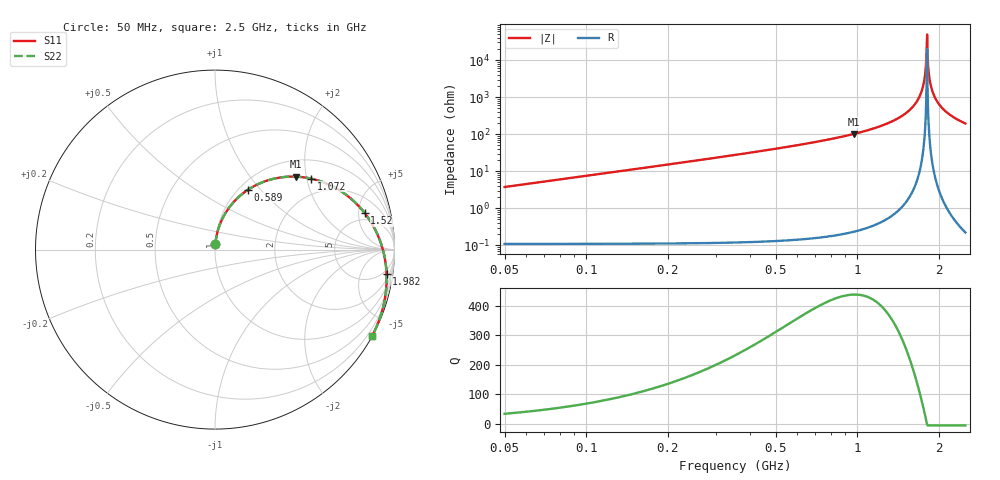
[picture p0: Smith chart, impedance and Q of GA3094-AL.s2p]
! Coilcraft GA3094-AL Air Core Inductor
! 01 July 2008
# MHZ S MA R 50
!Freq  MagS11  AngS11  MagS21  AngS21  MagS12  AngS12  MagS22  AngS22
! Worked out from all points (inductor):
!   351 points, 50 MHz to 2.5 GHz, reference 50 ohm
!   read as 1/Y11, port 2 shorted: L = 12 nH near 57 MHz
!   highest Q = 437 at 967 MHz (marker M1), where L = 16.7 nH
!   self-resonance near 1.8 GHz
!   S11 on the Smith chart (normalised r, x): 50 MHz: 1.00, +0.07; 589 MHz: 1.10, +0.86; 1.072 GHz: 1.50, +2.12; 1.52 GHz: 3.82, +5.92; 1.982 GHz: 3, -13; 2.5 GHz: 0.01, -3.91
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50  0.03286 85.7  0.9984 -2.4  0.9984 -2.4  0.03288 85.7
78  0.05124 85.0  0.9976 -3.8  0.9976 -3.8  0.05127 85.0
106  0.06962 84.0  0.9965 -5.1  0.9965 -5.1  0.06966 84.0
141  0.09258 82.5  0.9946 -6.8  0.9946 -6.8  0.09264 82.5
183  0.1201 80.6  0.9917 -8.9  0.9917 -8.9  0.1202 80.6
239  0.1568 78.0  0.9865 -11.6  0.9865 -11.6  0.1569 78.0
302  0.1979 75.0  0.9791 -14.6  0.9791 -14.6  0.198 75.0
463  0.3021 67.2  0.9521 -22.6  0.9521 -22.6  0.3023 67.2
589  0.3824 61.0  0.9228 -28.8  0.9228 -28.8  0.3826 61.0
869  0.5529 46.9  0.832 -43.0  0.832 -43.0  0.5532 46.9
967  0.6087 41.9  0.7921 -48.0  0.7921 -48.0  0.609 41.9
1072  0.6653 36.5  0.7452 -53.4  0.7452 -53.4  0.6657 36.5
1275  0.7636 26.0  0.6442 -63.9  0.6442 -63.9  0.764 26.0
1520  0.8589 13.7  0.5105 -76.2  0.5105 -76.2  0.8594 13.7
1688  0.9082 5.5  0.4165 -84.4  0.4165 -84.4  0.9087 5.5
1982  0.9652 -8.0  0.2589 -97.9  0.2589 -97.9  0.9657 -8.0
2094  0.9784 -12.8  0.2035 -102.7  0.2035 -102.7  0.9789 -12.8
2234  0.9896 -18.6  0.1391 -108.5  0.1391 -108.5  0.9902 -18.6
2346  0.9952 -23.0  0.09184 -112.8  0.09184 -112.8  0.9957 -23.0
2437  0.9978 -26.4  0.0563 -116.2  0.0563 -116.2  0.9984 -26.4
2472  0.9985 -27.7  0.04334 -117.5  0.04334 -117.5  0.999 -27.7
2500  0.9989 -28.7  0.03324 -118.5  0.03324 -118.5  0.9994 -28.7
